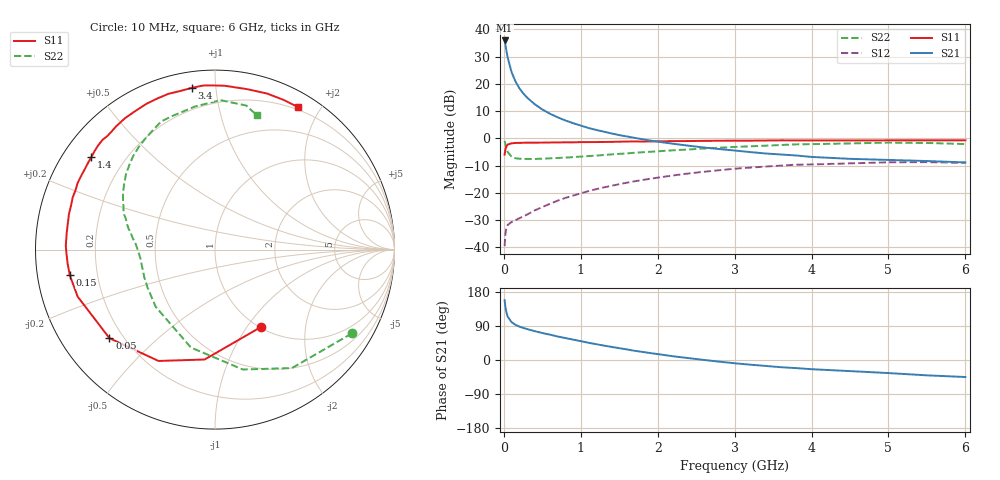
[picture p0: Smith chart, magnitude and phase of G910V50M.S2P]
! SIEMENS Small Signal Semiconductors
! BFG235
! Si NPN RF Bipolar Junction Transistor in SOT223
! VCE = 10 V  IC = 50 mA
! Common Emitter S-Parameters:  July  1994
# GHz  S  MA  R  50
!  f  S11  S21  S12  S22
! GHz  MAG  ANG  MAG  ANG  MAG  ANG  MAG  ANG
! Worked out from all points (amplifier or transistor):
!   40 points, 10 MHz to 6 GHz, reference 50 ohm
!   highest |S21| = 35.9 dB at 10 MHz (marker M1)
!   |S21| within 3 dB of that: start of sweep to 28.94 MHz
!   unconditionally stable (mu >= 1): 506.5 MHz to 1.365 GHz
!   at 200 MHz: K = 0.66, MSG = 23.9 dB, |S12| = -29.3 dB
!   at 1.5 GHz: K = 0.97, MSG = 9.0 dB, |S12| = -16.8 dB
!   at 6 GHz: K = 0.92, MSG = 0.1 dB, |S12| = -9.0 dB
!   S11 on the Smith chart (normalised r, x): 10 MHz: 1.01, -1.17; 50 MHz: 0.15, -0.36; 150 MHz: 0.10, -0.09; 1.4 GHz: 0.08, +0.33; 3.4 GHz: 0.08, +0.86; 6 GHz: 0.17, +1.73
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0.01  0.5016 -59.2  62.35 157.7  0.0105 69.4  0.8941 -31.5
0.02  0.6151 -95.4  52.26 140.7  0.0174 55.1  0.787 -57.0
0.03  0.6957 -116.9  43.27 128.6  0.0217 45.5  0.6859 -76.9
0.05  0.7677 -140.0  30.26 114.5  0.0258 34.9  0.562 -103.8
0.1  0.8088 -161.1  16.45 100.0  0.0291 30.5  0.459 -136.1
0.15  0.8215 -170.0  11.13 93.0  0.0313 33.7  0.4311 -150.5
0.2  0.8248 -174.6  8.351 88.4  0.0341 37.2  0.4233 -158.5
0.25  0.8278 -178.5  6.728 84.7  0.0367 40.8  0.418 -163.7
0.3  0.8316 178.6  5.625 81.8  0.0397 43.8  0.4174 -167.7
0.4  0.8314 173.7  4.232 76.1  0.0475 48.8  0.418 -172.6
0.5  0.8331 169.6  3.378 71.2  0.0547 52.1  0.4229 -176.2
0.6  0.8373 166.4  2.819 66.8  0.0629 54.1  0.4289 -179.2
0.7  0.839 162.8  2.426 62.1  0.0719 55.4  0.4357 178.2
0.9  0.8442 157.1  1.896 53.8  0.0888 55.7  0.4513 174.2
1.1  0.8516 150.6  1.546 45.4  0.1074 54.9  0.4722 170.1
1.4  0.8601 143.2  1.227 34.5  0.1345 52.0  0.5065 164.5
2.2  0.8874 124.4  0.794 9.8  0.2081 39.6  0.6026 148.3
3.2  0.9047 102.4  0.559 -12.3  0.2899 19.7  0.7126 126.5
3.4  0.9104 98.1  0.527 -15.6  0.3027 15.4  0.7319 121.7
4.5  0.9118 78.4  0.42 -29.3  0.3467 -6.8  0.8051 97.9
5.5  0.9175 65.2  0.383 -40.5  0.3653 -25.8  0.8212 77.7
6  0.9191 59.6  0.361 -44.9  0.3538 -32.6  0.7843 72.8
